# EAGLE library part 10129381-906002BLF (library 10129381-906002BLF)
Headers & Wire Housings ECONOSTIK HEADER DR VT TH 2X3 Source: Datasheet
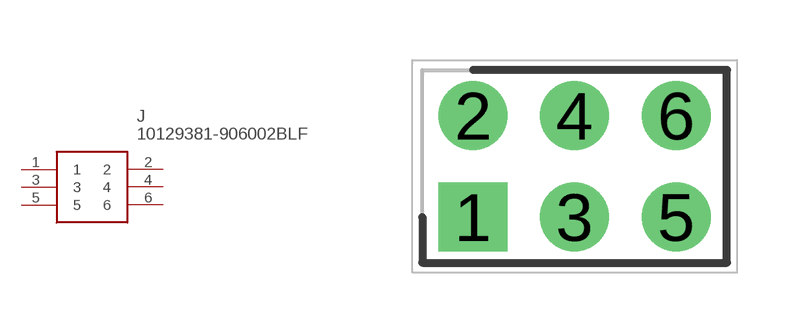
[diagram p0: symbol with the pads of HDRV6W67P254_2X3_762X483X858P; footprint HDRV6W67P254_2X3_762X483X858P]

Designator prefix J

## 10129381-906002BLF (Description: Headers & Wire Housings ECONOSTIK HEADER DR VT TH 2X3; Height: 8.58mm; Manufacturer_Name: Amphenol; Manufacturer_Part_Number: 10129381-906002BLF; Mouser_Part_Number: 649-1012938190602BLF; Mouser_Price-Stock: https://www.mouser.co.uk/ProductDetail/Amphenol-FCI/10129381-906002BLF/?qs=DXv0QSHKF4zSKXKyBbBVMw%3D%3D)  [HDRV6W67P254_2X3_762X483X858P]
1  1
2  2
3  3
4  4
5  5
6  6

## Footprint HDRV6W67P254_2X3_762X483X858P (pad centres in mm)
10129381-906002BLF
drill 1.15 pad 1.725 square: 1 0,0
drill 1.15 pad 1.725: 2 0,2.54; 3 2.54,0; 4 2.54,2.54; 5 5.08,0; 6 5.08,2.54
